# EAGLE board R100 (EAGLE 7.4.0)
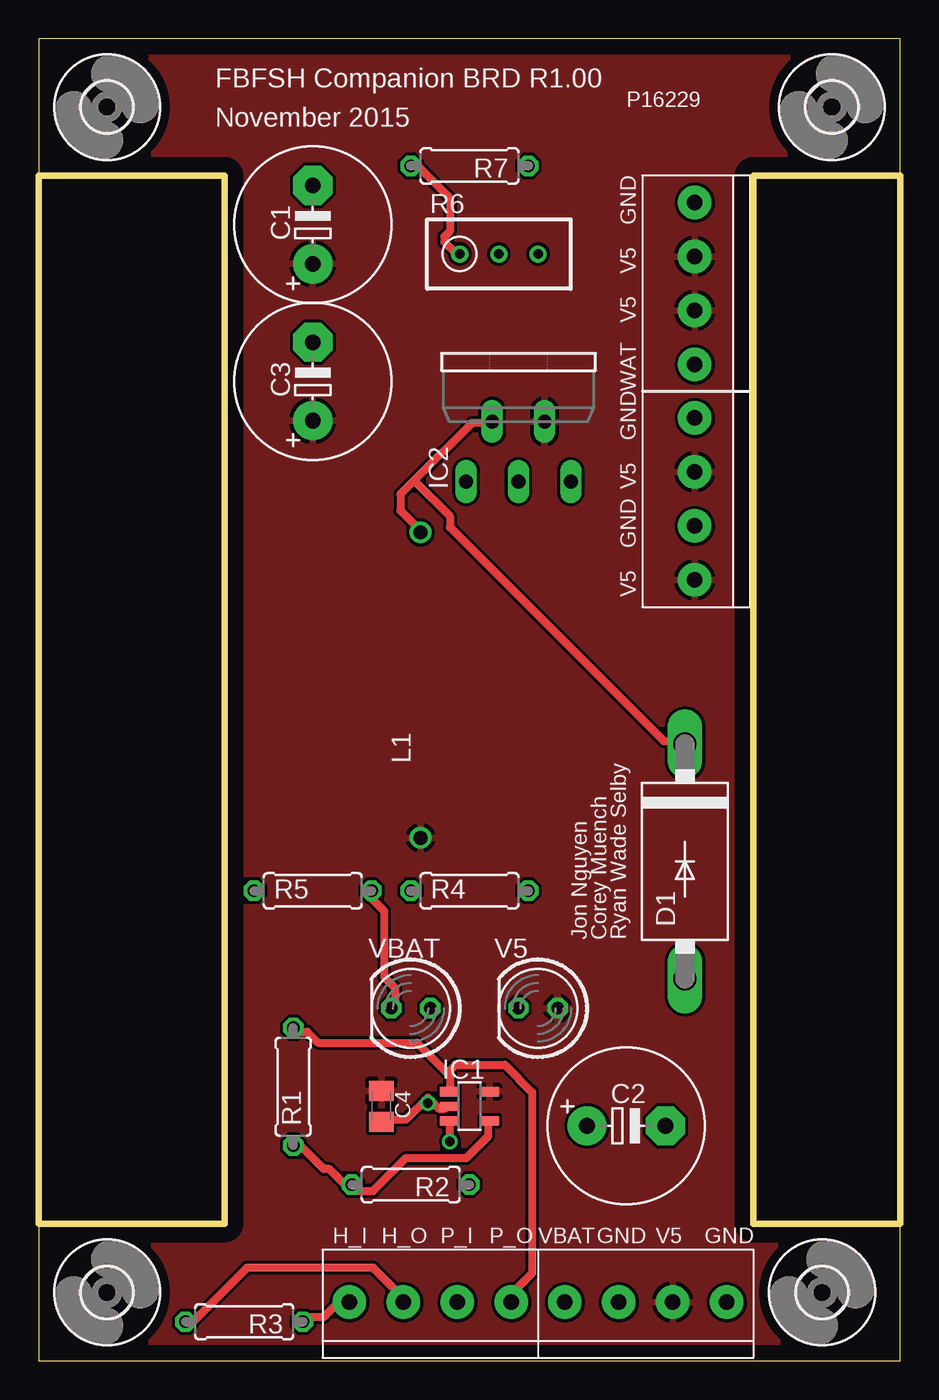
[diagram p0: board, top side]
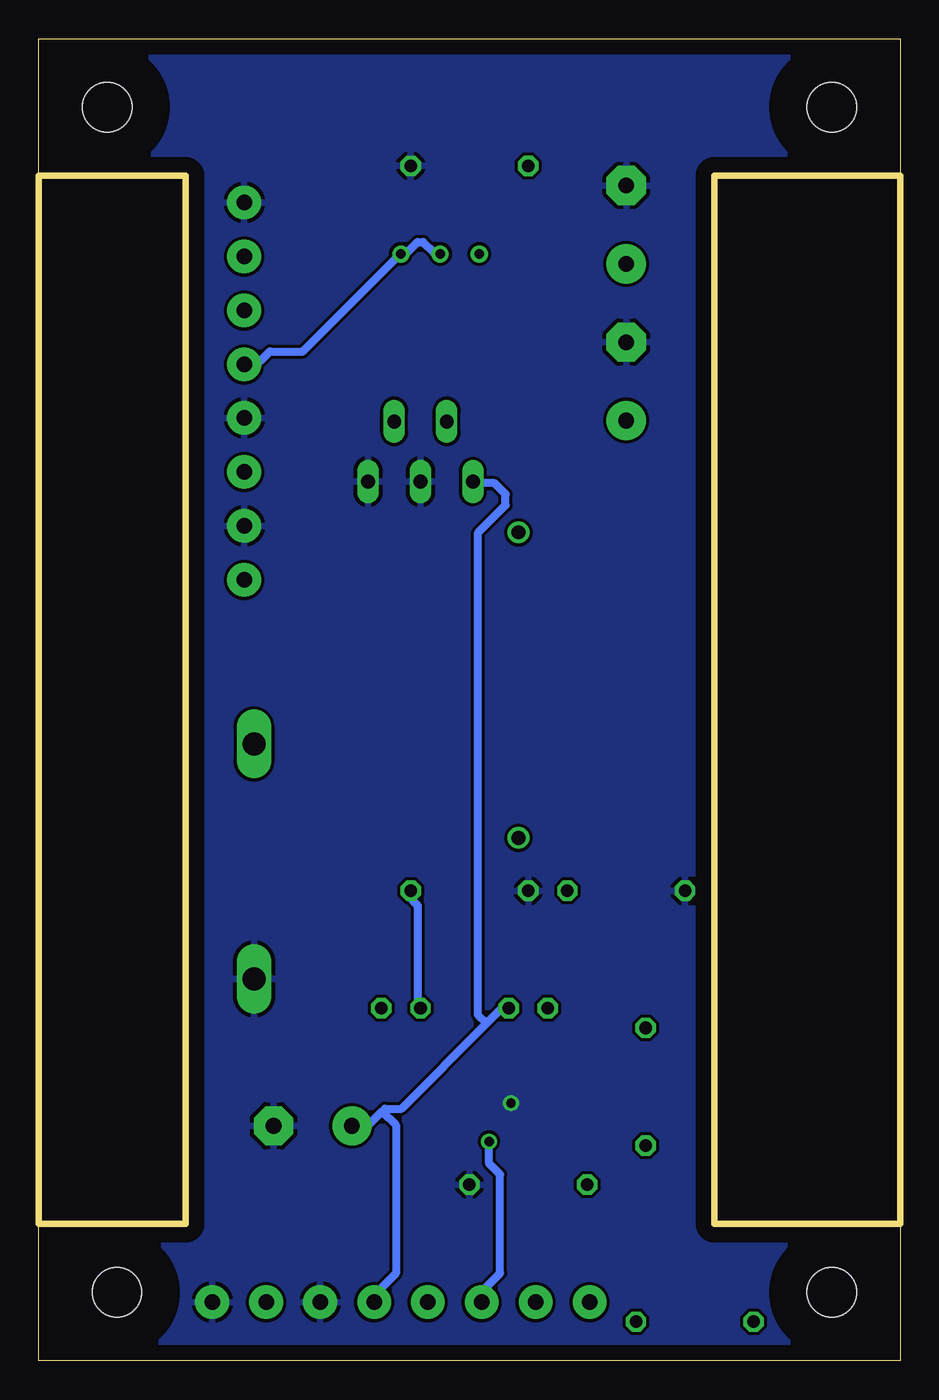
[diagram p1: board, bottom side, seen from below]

Size 55.88 x 85.72 mm. Coordinates in mm from the lower left corner, seen from the top.
Outline: 0,85.72 0,76.83 12.06,76.83 12.06,8.89 0,8.89 0,0 55.88,0 55.88,8.89 46.35,8.89 46.35,76.83 55.88,76.83 55.88,85.72 0,85.72
Copper layers (1*16): Top 0.035mm / dielectric 1.5mm / Bottom 0.035mm
Design rules "default": minimum track width 10mil, minimum drill 24mil, track to track 8mil, track to pad 8mil, pad to pad 8mil, via to via 8mil, smd to smd 8mil, copper to edge 40mil, drill to drill 8mil, minimum pad ring 10mil, minimum via ring 8mil, stop-mask expansion 4mil, vias tented up to drill 0mil, thermal gap 10mil
Net classes: 0 default: width 0.508 mm

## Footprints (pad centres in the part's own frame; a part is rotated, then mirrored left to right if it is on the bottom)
E5-10,5 = drill 1.016 pad 2.54: + -2.54,0 | drill 1.016 pad 2.54 octagon: - 2.54,0
C0805K = smd 1.3 x 1.6: 1 -1,0; 2 1,0
1X04-3.5MM = drill 1 pad 2.184: 1 -5.25,0; 2 -1.75,0; 3 1.75,0; 4 5.25,0
DO201-15 = drill 1.499 long: A 7.62,0; C -7.62,0
3,2 = hole 3.2: 0,0
SOT23-5 = smd 0.6 x 1.2: 1 -0.95,-1.306; 2 0,-1.306; 3 0.95,-1.306; 4 0.95,1.306; 5 -0.95,1.306
TO220-51 = drill 0.9 long: 1 -3.4,-8.4; 2 -1.7,-4.5; 3 0,-8.4; 4 1.7,-4.5; 5 3.4,-8.4
TJ4-U2 = drill 0.9: 1 -9.9,0; 2 9.9,0
0207/7 = drill 0.813 octagon: 1 -3.81,0; 2 3.81,0
RTRIM3296W = drill 0.61: 1 0,-2.54; 2 0,0; 3 0,2.54
LED5MM = drill 0.813 octagon: A -1.27,0; K 1.27,0

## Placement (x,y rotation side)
C1  1000uF  [E5-10,5]  17.78,73.66 90 top
C2  1000uF  [E5-10,5]  38.1,15.24 0 top
C3  1000uF  [E5-10,5]  17.78,63.5 90 top
C4  1uF  [C0805K]  22.23,16.51 270 top
CN1  1X4-3.5MM  [1X04-3.5MM]  39.37,3.81 0 top
CN2  1X4-3.5MM  [1X04-3.5MM]  25.4,3.81 0 top
CN3  1X4-3.5MM  [1X04-3.5MM]  42.55,69.85 90 top
CN4  1X4-3.5MM  [1X04-3.5MM]  42.55,55.88 90 top
D1  1N5822  [DO201-15]  41.91,32.38 270 top
H1  MOUNT-HOLE3.2  [3,2]  50.8,4.45 0 top
H2  MOUNT-HOLE3.2  [3,2]  4.45,4.45 0 top
H3  MOUNT-HOLE3.2  [3,2]  51.44,81.28 0 top
H4  MOUNT-HOLE3.2  [3,2]  4.45,81.28 0 top
IC1  TS931ILT  [SOT23-5]  27.94,16.51 270 top
IC2  LM2576T-005G  [TO220-51]  31.11,65.41 0 top
L1  150uF  [TJ4-U2]  24.77,43.81 90 top
R1  124K  [0207/7]  16.51,17.78 90 top
R2  1K  [0207/7]  24.13,11.43 180 top
R3  1K  [0207/7]  13.34,2.54 180 top
R4  150  [0207/7]  27.94,30.48 0 top
R5  1K  [0207/7]  17.78,30.48 0 top
R6  500K  [RTRIM3296W]  29.84,71.75 270 top
R7  500K  [0207/7]  27.94,77.47 180 top
V5  RED  [LED5MM]  32.38,22.86 180 top
VBAT  BLUE  [LED5MM]  24.13,22.86 180 top

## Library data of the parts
C1-C4 L1 R1-R7 = resistor
CN1-CN4 = adafruit
D1 = diode
H1-H4 = holes
IC1 IC2 = linear
V5 VBAT = led

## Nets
GND: C1.- C2.- C3.- C4.2 CN1.2 CN1.4 CN3.4 CN4.2 CN4.4 D1.A IC1.2 IC2.3 IC2.5 R2.1 R4.1 R5.1 R7.1
H_IN: CN2.1 R3.1
H_OUT: CN2.2 R3.2
N$1: R6.1 R7.2
N$2: IC1.4 R1.1 R2.2
N$4: R4.2 V5.K
N$5: D1.C IC2.2 L1.2
N$6: R5.2 VBAT.K
P_IN: CN2.3 IC1.3
P_OUT: CN2.4 IC1.1 R1.2
V5: C1.+ C3.+ C4.1 CN1.3 CN3.2 CN3.3 CN4.1 CN4.3 IC1.5 IC2.4 L1.1 V5.A
VBST: C2.+ CN1.1 IC2.1 VBAT.A
WAT: CN3.1 R6.2 R6.3

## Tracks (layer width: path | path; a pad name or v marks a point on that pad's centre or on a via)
GND  (via drill 0.61)
  Top 0.508: 25.43,16.89 25.25,17.07 23.82,15.65 22.4,15.65 C4.2 | 25.43,16.89 25.96,16.36 26.31,16.36 IC1.2 | v25.25,16.71 25.43,16.89
  pour Bottom: 0,0 55.88,0 55.88,8.89 46.35,8.89 46.35,76.83 55.88,76.83 55.88,85.72 0,85.72 0,76.83 12.06,76.83 12.06,8.89 0,8.89
H_IN
  Top 0.508: R3.1 17.42,2.85 18.49,2.85 19.2,3.56 19.91,3.56 CN2.1
H_OUT
  Top 0.508: R3.2 9.6,2.49 9.96,2.49 13.51,6.04 21.69,6.04 23.82,3.91 CN2.2
N$1
  Top 0.508: R6.1 27.03,71.83 26.31,72.54 26.31,72.9 26.67,73.25 26.67,75.39 24.54,77.52 24.18,77.52 R7.2
N$2
  Top 0.508: 20.27,11.02 21.69,11.02 23.82,13.16 27.74,13.16 29.16,14.58 29.16,15.29 IC1.4 | 20.27,11.02 20.27,11.38 R2.2 20.27,11.02 | 20.27,11.02 18.85,12.45 18.49,12.45 17.07,13.87 16.71,13.87 R1.1
N$4
  Bottom 0.508: V5.K 31.29,23.11 31.29,29.52 32,30.23 R4.2
N$5
  Top 0.508: 24.36,57.07 28.09,60.81 29.16,60.81 IC2.2 | 24.36,57.07 23.47,56.19 23.47,55.12 24.54,54.05 L1.2 | 24.36,57.07 26.67,54.76 26.67,54.05 40.54,40.18 41.6,40.18 D1.C
N$6
  Top 0.508: VBAT.K 23.11,23.11 23.11,24.18 22.4,24.89 22.4,29.16 21.34,30.23 R5.2
P_IN  (via drill 0.61)
  Top 0.508: v26.67,14.22 26.67,15.29 IC1.3
  Bottom 0.508: v26.67,14.22 26.67,12.8 25.96,12.09 25.96,5.69 27.03,4.62 27.03,3.91 CN2.3
P_OUT
  Top 0.508: 26.49,18.67 24.54,20.62 18.14,20.62 17.42,21.34 16.71,21.34 R1.2 | 26.49,18.67 26.67,18.49 26.67,17.42 IC1.1 | 26.49,18.67 27.03,19.2 30.23,19.2 32,17.42 32,5.69 30.94,4.62 30.94,3.91 CN2.4
V5
  pour Top: 0,85.72 55.88,85.72 55.88,76.83 46.35,76.83 46.35,8.89 55.88,8.89 55.88,0 0,0 0,8.89 12.06,8.89 12.06,76.83 0,76.83
VBST
  Bottom 0.508: 26.85,21.87 32.36,16.36 33.43,16.36 33.6,16.18 | 26.85,21.87 25.96,22.76 25.6,22.76 VBAT.A | 33.6,16.18 34.49,15.29 35.56,15.29 C2.+ | 26.85,21.87 27.38,22.4 27.38,53.7 25.6,55.47 25.6,56.19 26.31,56.9 27.38,56.9 IC2.1 | 33.6,16.18 32.72,15.29 32.72,5.69 33.78,4.62 33.78,3.91 CN1.1
WAT
  Bottom 0.508: R6.2 29.87,71.83 30.23,71.83 30.94,72.54 31.29,72.54 32.36,71.48 R6.3 32.72,71.48 38.76,65.43 40.89,65.43 41.6,64.72 42.32,64.72 CN3.1

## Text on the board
tNames: FBFSH Companion BRD R1.00 | P16229 | November 2015 | GND | V5 | V5 | WAT | GND | V5 | GND | V5 | Jon Nguyen | Corey Muench | Ryan Wade Selby | H_I | H_O | P_I | P_O | VBAT | GND | V5 | GND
